FUNCTION_BLOCK p08_ST_materialTracking
VAR_INPUT
END_VAR
VAR_OUTPUT
END_VAR
VAR
	location: ARRAY[0..7] OF ST_LOCATION;
END_VAR

location[0].occupied := TRUE;
location[0].workpiece.id := 42;
location[0].workpiece.recipe.directionMachine1 := FALSE;
location[0].workpiece.recipe.timeMachine1 := T#1S;
location[0].workpiece.recipe.positionSequence[0].rotation := 100;
location[0].workpiece.recipe.positionSequence[0].lift := 50;
location[0].workpiece.recipe.positionSequence[0].extension := 30;
location[0].workpiece.recipe.positionSequence[0].grip := 15;

// Trasnsfer of material forward
IF location[0].isDone THEN
	location[1].workpiece := location[0].workpiece;
	location[0].isDone := FALSE;
END_IF

END_FUNCTION_BLOCK
